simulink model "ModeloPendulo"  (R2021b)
settings: Solver=ode3  StartTime=0.0  StopTime=20  FixedStep=1e-3  RelTol=1e-3  EnableMultiTasking=on
InitFcn:
  | linear = readfis('linear.fis');
  | 
  | 
  | Rm = 8.7;
  | Kt = 0.03334;
  | Km = 0.03334;
  | Jm = 1.8e-6;
  | Jeq = 1.84e-4;
  | Marm = 0.08;
  | r = 0.0826;
  | Beq = 4.7940e-03;
  | Mp = 0.0270;
  | lp = 0.153;
  | Jp = 1.7e-4;
  | Bp = 0;
  | g = 9.81;
  | 
  | a = Jeq + (Mp*r*r);
  | b = Mp*lp*r;
  | c = Jp + (Mp*lp*lp);
  | d = Mp*g*lp;
  | G = (Kt*Km)/Rm;

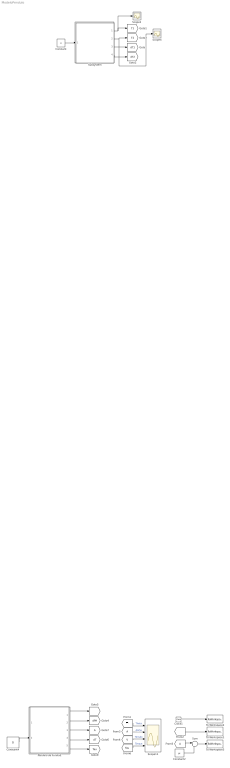
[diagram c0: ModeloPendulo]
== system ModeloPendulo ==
  Clock1 : Clock
  Constant : Constant  Commented=on  Value=0
  Constant2 : Constant  Value=pi
  Constant4 : Constant  Value=0
  From3 : From  TagVisibility=global
  From5 : From  TagVisibility=global
  Goto7 : Goto  TagVisibility=global
  Pêndulo de Furuta2 : Subsystem
  Scope11 : Scope  NumInputPorts=4
  Scope2 : Scope
  Scope4 : Scope
  Subsystem : Subsystem  Commented=on
  Sum : Sum  Inputs=|+-
  To Workspace1 : ToWorkspace  VariableName=simTheta  SampleTime=-1
  To Workspace2 : ToWorkspace  VariableName=simt  SampleTime=-1
  To Workspace3 : ToWorkspace  VariableName=simAlpha  SampleTime=-1
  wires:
  Constant/1 -> Subsystem/1(E)
  Subsystem/2(T2) -> Scope4/1, [T2]
  Subsystem/4(dT2) -> [dT2]
  Subsystem/3(dT1) -> [dT1]
  Subsystem/1(T1) -> Scope2/1, [T1]
  Clock1/1 -> To Workspace2/1
  Constant2/1 -> Sum/2
  Pêndulo de Furuta2/3(Alfa.) -> Goto7/1
  Pêndulo de Furuta2/1(Theta.) -> [T]
  Pêndulo de Furuta2/2(dTheta.) -> [dPH]
  Pêndulo de Furuta2/4(dAlfa.) -> [dT]
  [T] -> Scope11/1  "Theta"
  From3/1 -> Scope11/2  "Alpha"
  [V] -> Scope11/3  "Tensão"
  Constant4/1 -> Pêndulo de Furuta2/2(Alfa (0))
  [T] -> To Workspace1/1
  From5/1 -> Sum/1
  Sum/1 -> To Workspace3/1
  [Tau] -> Scope11/4  "Torque"
  Pêndulo de Furuta2/5(Tau) -> [Tau]

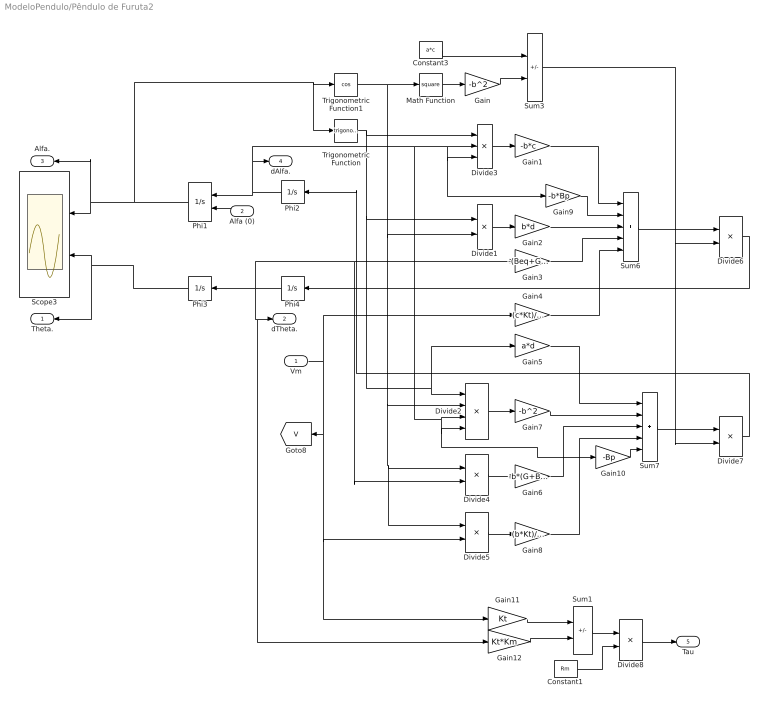
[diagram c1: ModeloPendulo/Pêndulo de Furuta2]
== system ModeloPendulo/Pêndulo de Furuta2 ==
  Vm : Inport
  Alfa (0) : Inport  Port=2
  Constant1 : Constant  Value=Rm
  Constant3 : Constant  Value=a*c
  Divide1 : Product  Inputs=**
  Divide2 : Product  Inputs=****
  Divide3 : Product  Inputs=***
  Divide4 : Product  Inputs=**
  Divide5 : Product  Inputs=**
  Divide6 : Product  Inputs=*/
  Divide7 : Product  Inputs=*/
  Divide8 : Product  Inputs=*/
  Gain : Gain  Gain=-b^2
  Gain1 : Gain  Gain=-b*c
  Gain10 : Gain  Gain=-Bp
  Gain11 : Gain  Gain=Kt
  Gain12 : Gain  Gain=Kt*Km
  Gain2 : Gain  Gain=b*d
  Gain3 : Gain  Gain=-(Beq+G)*c
  Gain4 : Gain  Gain=(c*Kt)/Rm
  Gain5 : Gain  Gain=a*d
  Gain6 : Gain  Gain=-b*(G+Beq)
  Gain7 : Gain  Gain=-b^2
  Gain8 : Gain  Gain=(b*Kt)/Rm
  Gain9 : Gain  Gain=-b*Bp
  Math Function : Math  Operator=square  SignedPower=on
  Phi1 : Integrator  InitialConditionSource=external
  Phi2 : Integrator
  Phi3 : Integrator
  Phi4 : Integrator
  Scope3 : Scope  NumInputPorts=2
  Sum1 : Sum  Inputs=+-
  Sum3 : Sum  Inputs=+-
  Sum6 : Sum  Inputs=+++++
  Sum7 : Sum  Inputs=+++++
  Trigonometric Function : Trigonometry
  Trigonometric Function1 : Trigonometry  Operator=cos
  Theta. : Outport
  dTheta. : Outport  Port=2
  Alfa. : Outport  Port=3
  dAlfa. : Outport  Port=4
  Tau : Outport  Port=5
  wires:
  Phi1/1 -> Alfa./1, Scope3/1, Trigonometric Function/1, Trigonometric Function1/1
  Phi4/1 -> Gain12/1, dTheta./1, Divide4/2, Gain3/1, Phi3/1
  Phi3/1 -> Theta./1, Scope3/2
  Trigonometric Function1/1 -> Math Function/1, Divide1/2, Divide2/2, Divide5/1, Divide4/1
  Math Function/1 -> Gain/1
  Constant3/1 -> Sum3/1
  Trigonometric Function/1 -> Divide3/1, Divide1/1, Gain5/1, Divide2/1
  Gain/1 -> Sum3/2
  Divide3/1 -> Gain1/1
  Divide1/1 -> Gain2/1
  Gain4/1 -> Sum6/5
  Gain3/1 -> Sum6/4
  Gain2/1 -> Sum6/3
  Gain1/1 -> Sum6/1
  Divide2/1 -> Gain7/1
  Divide4/1 -> Gain6/1
  Vm/1 -> [V], Gain11/1, Divide5/2, Gain4/1
  Divide5/1 -> Gain8/1
  Gain8/1 -> Sum7/4
  Gain5/1 -> Sum7/1
  Gain7/1 -> Sum7/2
  Gain6/1 -> Sum7/3
  Sum6/1 -> Divide6/1
  Sum7/1 -> Divide7/1
  Sum3/1 -> Divide7/2, Divide6/2
  Divide6/1 -> Phi4/1
  Divide7/1 -> Phi2/1
  Phi2/1 -> dAlfa./1, Gain10/1, Divide2/4, Divide2/3, Gain9/1, Divide3/3, Divide3/2, Phi1/1
  Gain9/1 -> Sum6/2
  Gain10/1 -> Sum7/5
  Alfa (0)/1 -> Phi1/2
  Gain11/1 -> Sum1/1
  Gain12/1 -> Sum1/2
  Sum1/1 -> Divide8/1
  Divide8/1 -> Tau/1
  Constant1/1 -> Divide8/2

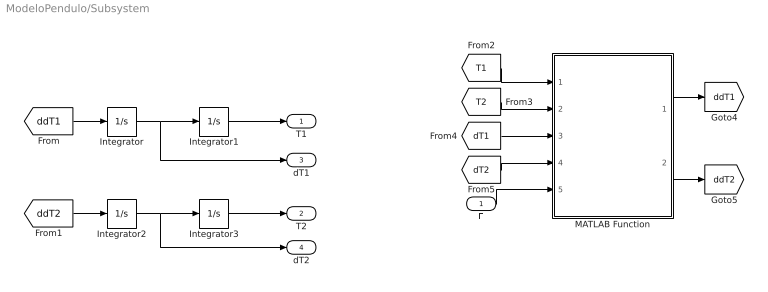
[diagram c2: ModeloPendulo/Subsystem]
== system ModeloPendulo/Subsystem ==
  E : Inport
  Integrator : Integrator  InitialCondition=0.0001
  Integrator1 : Integrator
  Integrator2 : Integrator
  Integrator3 : Integrator
  MATLAB Function : MATLAB Function  TreatAsAtomicUnit=on
  T1 : Outport
  T2 : Outport  Port=2
  dT1 : Outport  Port=3
  dT2 : Outport  Port=4
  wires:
  E/1 -> MATLAB Function/5(E)
  Integrator3/1 -> T2/1
  MATLAB Function/2(ddT2) -> [ddT2]
  [dT2] -> MATLAB Function/4(dT2)
  MATLAB Function/1(ddT1) -> [ddT1]
  Integrator/1 -> dT1/1, Integrator1/1
  Integrator1/1 -> T1/1
  Integrator2/1 -> dT2/1, Integrator3/1
  [ddT1] -> Integrator/1
  [ddT2] -> Integrator2/1
  [T1] -> MATLAB Function/1(T1)
  [T2] -> MATLAB Function/2(T2)
  [dT1] -> MATLAB Function/3(dT1)

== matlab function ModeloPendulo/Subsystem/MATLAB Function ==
function [ddT1,ddT2] = fcn(T1,T2,dT1,dT2,E)


%Carregando variáveis
m1 = 0.065;
m2 = 0.022;
L1 = 0.14;
c2 = 0.156;
J1 = 1.569e-3;
J2 = 1.746e-4;
g = 9.81;
Ra = 1.0827;
Kb = 0.01376;
Kt = 0.01376;


%Matrizes
M11 = J1 + m2*L1^2 + (m2*c2^2 + J2)*sin(T2)^2;
M12 = m2*L1*c2*cos(T2);
M21 = m2*L1*c2*cos(T2);
M22 = m2*c2^2 + J2;
M = [M11 M12; M21 M22];

C11 = (m2*c2^2 + J2)*dT1*dT2*sin(2*T2) - m2*L1*c2*dT2^2*sin(T2);
C21 = -0.5*m2*c2^2*dT1^2*sin(2*T2);
C = [C11; C21];

G11 = (Kt*Kb)/(Ra*dT1);
G21 = -m2*g*c2*sin(T2);
G = [G11; G21];

V11 = Kt/Ra;
V21 = 0;
V = [V11; V21];

%Equação dinâmica
T = inv(M)*(-C-G+V*E);
ddT1 = T(1,1);
ddT2 = T(2,1);
end
